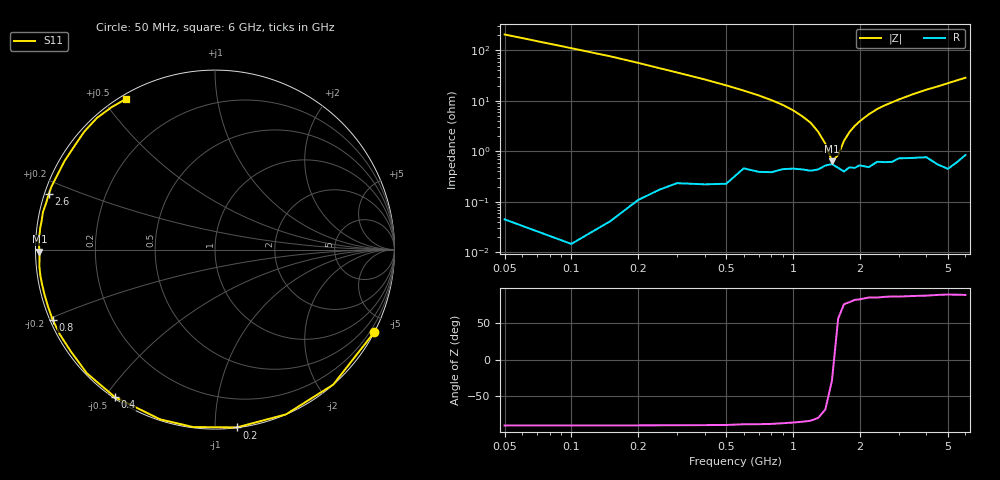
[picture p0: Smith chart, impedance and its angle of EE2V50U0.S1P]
! Infineon Technologies  Discrete & RF Semiconductors
! BBY55-02W
! Si Tuning Diode in SCD-80
! VR = 2.5 V
! S-Parameters:  June  2000
# GHz  S  MA  R  50
!  f  S11
! GHz  MAG  ANG
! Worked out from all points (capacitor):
!   34 points, 50 MHz to 6 GHz, reference 50 ohm
!   read as one part to ground: C = 14.4 pF near 50 MHz
!   lowest |Z| = 637 mohm at 1.5 GHz (marker M1)
!   series resonance near 1.53 GHz, so ESL is about 750 pH
!   S11 on the Smith chart (normalised r, x): 50 MHz: 0.00, -4.12; 200 MHz: 0.00, -1.13; 400 MHz: 0.00, -0.53; 800 MHz: 0.01, -0.21; 2.6 GHz: 0.01, +0.16; 6 GHz: 0.02, +0.57
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0.05  0.9999 -27.3
0.1  0.9999 -48.8
0.15  0.9995 -66.7
0.2  0.9981 -83.0
0.25  0.9961 -97.0
0.3  0.9939 -107.9
0.4  0.9931 -124.2
0.5  0.9922 -136.0
0.6  0.9834 -144.7
0.7  0.9854 -151.3
0.8  0.9853 -156.7
0.9  0.9829 -161.2
1  0.9823 -165.2
1.1  0.9828 -168.7
1.3  0.9827 -174.5
1.5  0.9779 -179.3
1.6  0.9814 178.4
1.7  0.9842 176.4
2.2  0.981 167.7
2.4  0.9759 164.4
2.6  0.9765 161.5
2.8  0.9764 158.9
3.5  0.9728 149.5
4  0.9728 143.3
4.5  0.9811 137.9
5  0.9851 131.9
5.5  0.9808 126.1
6  0.9749 120.4
